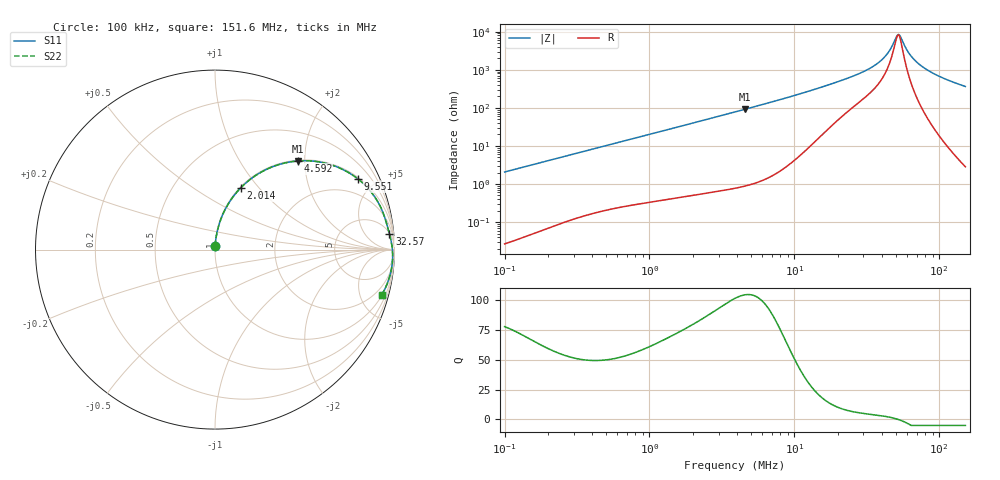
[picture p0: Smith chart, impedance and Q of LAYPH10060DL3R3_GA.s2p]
! LAYPH10060DL3R3_GA  S-PARAMETER MODEL  ( General Type )
! Model Generated by TAIYO YUDEN Corporation (http://www.ty-top.com)
! Version 3.0
! TAIYO YUDEN Control No. 180828NI43SB-FBB
! Copyright(c) 2017 TAIYO YUDEN CO.,LTD. All Rights Reserved.
! Product Description (link to TY-COMPAS)
! https://ds.yuden.co.jp/TYCOMPAS/or/detail?pn=LAYPH10060DL3R3NGA&u=M
! Products Name : Inductors
! Characteristics :
!  Inductance : 3.3 uH , SRF(min) : -Hz , DC Resistance(max) : 0.012 Ohm
!  Rated Current : Saturation :7 A , Temp Rise : 4.7 A (25 degC)
!  Case Size : 10.1 x 10.0 / 0.398 x 0.394 [mm/inch] , Thickness : 6 / 0.236 [mm/inch]
!  (Conditions: Temperature = 25 degC , DC Bias Current/Voltage = 0A / 0V)
! External Node Assignments :
!  1  o---GGG---o  2
! GND o---------o GND
! Frequency Range : 0.1MHz  -  151.640846MHz  [ 402 STEP ]
# MHz S RI R 50
! Freq[MHz].  S11 Real  S11 Imag  S21 Real  S21 Imag  S12 Real  S12 Imag  S22 Real  S22 Imag
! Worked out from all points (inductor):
!   401 points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, 100 kHz to 151.6 MHz, reference 50 ohm
!   read as one part in series: L = 3.29 uH near 103.7 kHz
!   highest Q = 104 at 4.592 MHz (marker M1), where L = 3.2 uH
!   self-resonance near 51.48 MHz
!   S11 on the Smith chart (normalised r, x): 100 kHz: 1.00, +0.04; 2.014 MHz: 1.01, +0.81; 4.592 MHz: 1.02, +1.85; 9.551 MHz: 1.07, +4.01; 32.57 MHz: 6, +20; 151.6 MHz: 1.06, -7.28
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0.1  0.000693 0.0206  0.9993 -0.0206  0.9993 -0.0206  0.000693 0.0206
0.341025  0.00619 0.0691  0.9938 -0.0691  0.9938 -0.0691  0.00619 0.0691
1.162983  0.0546 0.2197  0.9454 -0.2197  0.9454 -0.2197  0.0546 0.2197
2.014349  0.1427 0.3435  0.8573 -0.3435  0.8573 -0.3435  0.1427 0.3435
3.894109  0.38 0.4805  0.62 -0.4805  0.62 -0.4805  0.38 0.4805
4.591731  0.4608 0.4937  0.5392 -0.4937  0.5392 -0.4937  0.4608 0.4937
6.502274  0.6355 0.476  0.3645 -0.476  0.3645 -0.476  0.6355 0.476
9.551203  0.7962 0.3939  0.2038 -0.3939  0.2038 -0.3939  0.7962 0.3939
13.2799  0.8862 0.2993  0.1138 -0.2993  0.1138 -0.2993  0.8862 0.2993
23.00149  0.9527 0.157  0.0473 -0.157  0.0473 -0.157  0.9527 0.157
32.57203  0.9715 0.0889  0.0285 -0.0889  0.0285 -0.0889  0.9715 0.0889
39.83981  0.9804 0.0517  0.0196 -0.0517  0.0196 -0.0517  0.9804 0.0517
45.28783  0.9849 0.0274  0.0151 -0.0274  0.0151 -0.0274  0.9849 0.0274
50.54681  0.9877 0.00604  0.0123 -0.00604  0.0123 -0.00604  0.9877 0.00604
52.43217  0.9884 -0.00123  0.0116 0.00123  0.0116 0.00123  0.9884 -0.00123
54.38786  0.9889 -0.00858  0.0111 0.00858  0.0111 0.00858  0.9889 -0.00858
59.60218  0.9898 -0.0273  0.0102 0.0273  0.0102 0.0273  0.9898 -0.0273
62.96776  0.9898 -0.0388  0.0102 0.0388  0.0102 0.0388  0.9898 -0.0388
69.00467  0.9891 -0.0583  0.0109 0.0583  0.0109 0.0583  0.9891 -0.0583
75.62035  0.9874 -0.0785  0.0126 0.0785  0.0126 0.0785  0.9874 -0.0785
101.3611  0.9738 -0.1474  0.0262 0.1474  0.0262 0.1474  0.9738 -0.1474
151.6408  0.9281 -0.2544  0.0719 0.2544  0.0719 0.2544  0.9281 -0.2544
